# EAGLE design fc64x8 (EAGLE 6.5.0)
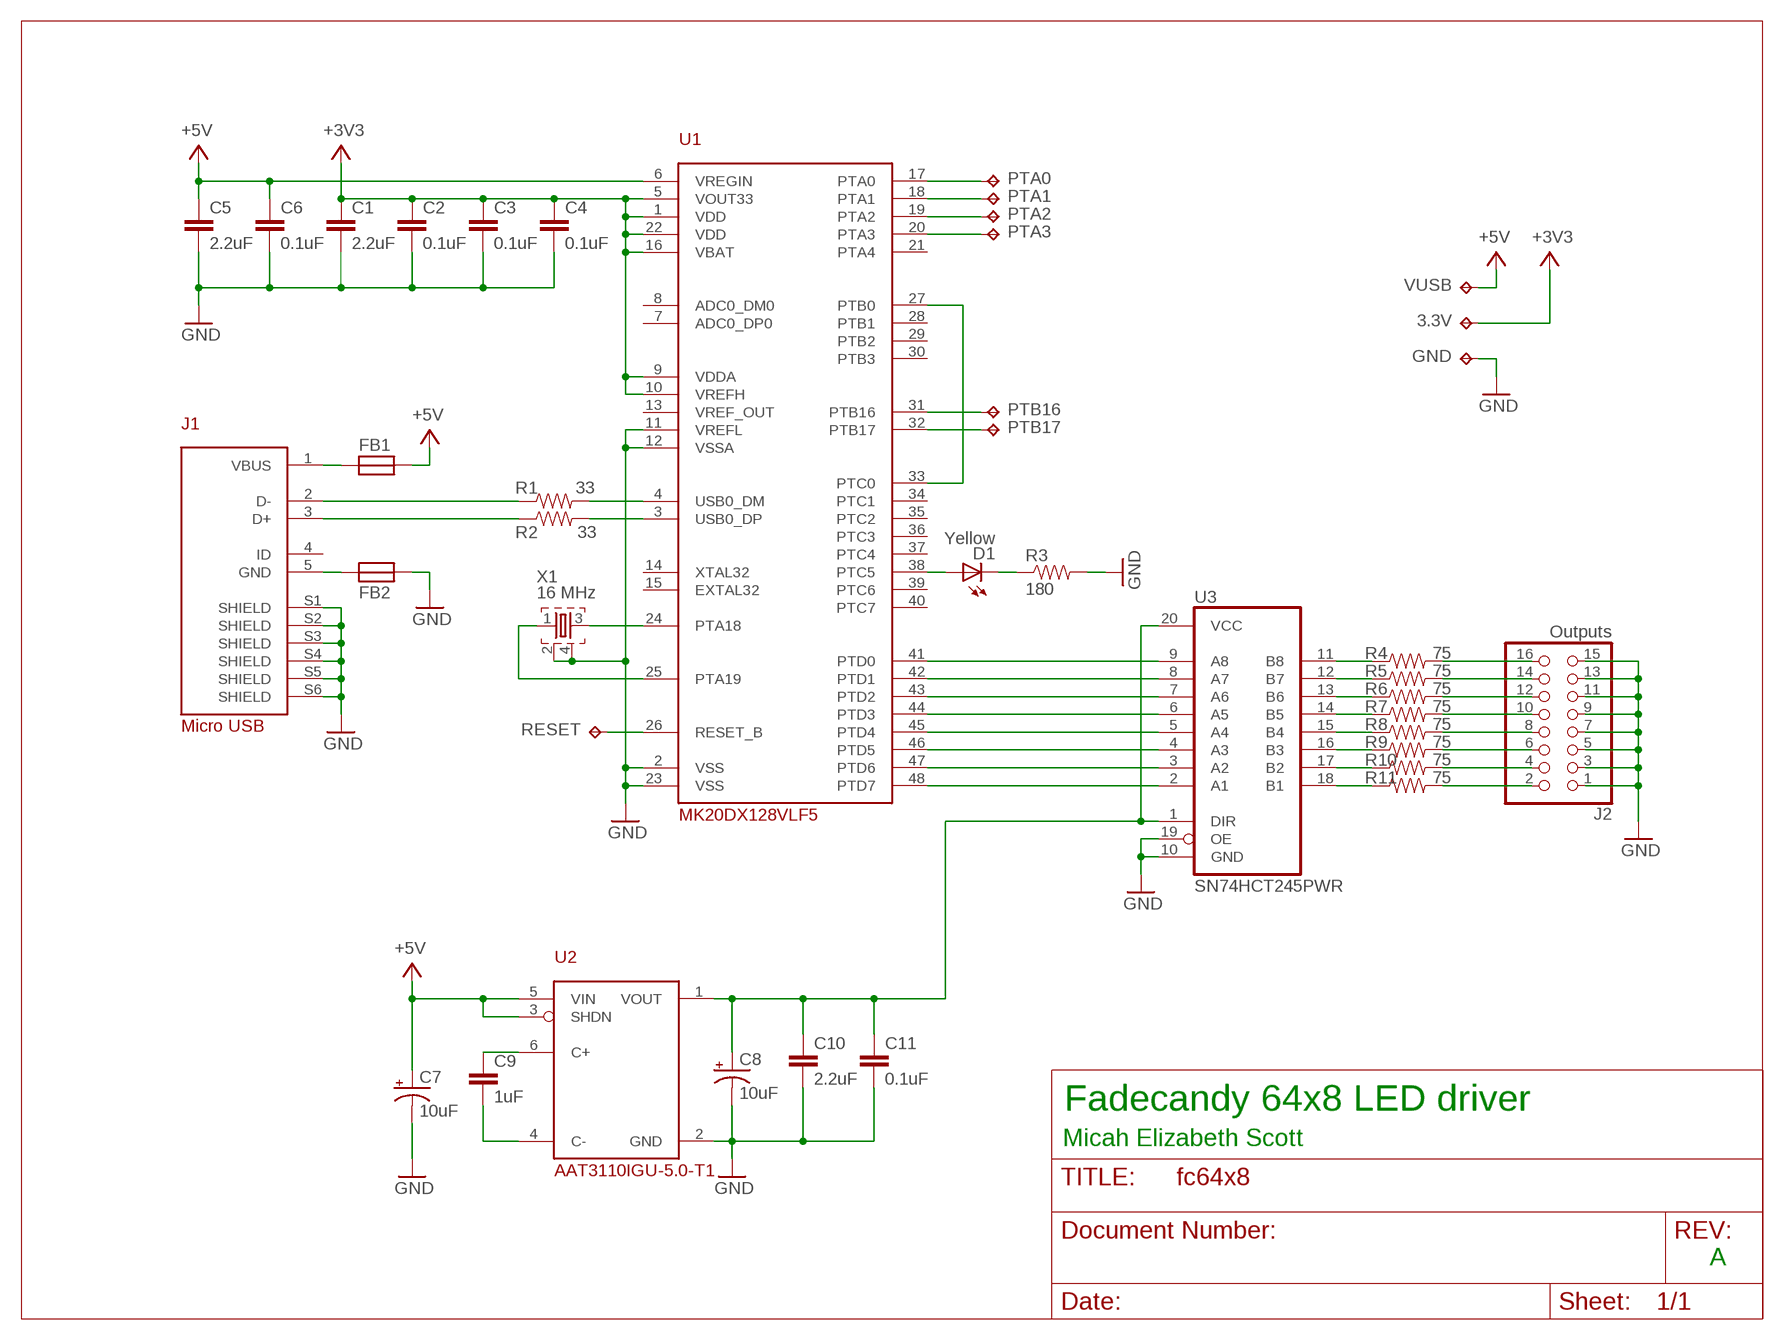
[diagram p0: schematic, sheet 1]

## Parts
3.3V  TPTP18SQ  [TP18SQ]
C1  2.2uF  CAP0603-CAP  [0603-CAP]
C2  0.1uF  CAP0603-CAP  [0603-CAP]
C3  0.1uF  CAP0603-CAP  [0603-CAP]
C4  0.1uF  CAP0603-CAP  [0603-CAP]
C5  2.2uF  CAP0603-CAP  [0603-CAP]
C6  0.1uF  CAP0603-CAP  [0603-CAP]
C7  10uF  CAP_POL1206  [EIA3216]
C8  10uF  CAP_POL1206  [EIA3216]
C9  1uF  CAP0603-CAP  [0603-CAP]
C10  2.2uF  CAP0603-CAP  [0603-CAP]
C11  0.1uF  CAP0603-CAP  [0603-CAP]
D1  Yellow  LED-YELLOW0603  [LED-0603]
FB1  FB  [0603]
FB2  FB  [0603]
GND  TPTP18SQ  [TP18SQ]
J1  Micro USB  USB-FCI-10118194  [FCI-10118194]
J2  Outputs  PINHD-2X8  [2X08]
PTA0  TPTP18SQ  [TP18SQ]
PTA1  TPTP18SQ  [TP18SQ]
PTA2  TPTP18SQ  [TP18SQ]
PTA3  TPTP18SQ  [TP18SQ]
PTB16  TPTP18SQ  [TP18SQ]
PTB17  TPTP18SQ  [TP18SQ]
R1  33  RESISTOR0603-RES  [0603-RES]
R2  33  RESISTOR0603-RES  [0603-RES]
R3  180  RESISTOR0603-RES  [0603-RES]
R4  75  RESISTOR0603-RES  [0603-RES]
R5  75  RESISTOR0603-RES  [0603-RES]
R6  75  RESISTOR0603-RES  [0603-RES]
R7  75  RESISTOR0603-RES  [0603-RES]
R8  75  RESISTOR0603-RES  [0603-RES]
R9  75  RESISTOR0603-RES  [0603-RES]
R10  75  RESISTOR0603-RES  [0603-RES]
R11  75  RESISTOR0603-RES  [0603-RES]
RESET  TPTP18SQ  [TP18SQ]
U1  MK20DX128VLF5  [LQFP48]
U2  AAT3110IGU-5.0-T1  AAT3110  [SOT23-6L]
U3  SN74HCT245PWR  74245PW  [TSSOP20]
VUSB  TPTP18SQ  [TP18SQ]
X1  16 MHz  TSX-32250  [TSX-3225]

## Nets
+3V3: 3.3V.TP C1.1 C2.1 C3.1 C4.1 U1.1(VDD) U1.5(VOUT33) U1.9(VDDA) U1.10(VREFH) U1.16(VBAT) U1.22(VDD)
+5V: C5.1 C6.1 C7.A(+) FB1.1 U1.6(VREGIN) U2.3(SHDN) U2.5(VIN) VUSB.TP
GND: C1.2 C2.2 C3.2 C4.2 C5.2 C6.2 C7.C(-) C8.C(-) C10.2 C11.2 FB2.1 GND.TP J1.S1(SHIELD) J1.S2(SHIELD) J1.S3(SHIELD) J1.S4(SHIELD) J1.S5(SHIELD) J1.S6(SHIELD) J2.1 J2.3 J2.5 J2.7 J2.9 J2.11 J2.13 J2.15 R3.2 U1.2(VSS) U1.11(VREFL) U1.12(VSSA) U1.23(VSS) U2.2(GND) U3.10(GND) U3.19(OE) X1.2 X1.4
N$1: D1.A U1.38(PTC5)
N$2: U1.24(PTA18) X1.3
N$3: D1.C R3.1
N$4: U1.25(PTA19) X1.1
N$5: FB1.2 J1.1(VBUS)
N$6: U1.27(PTB0) U1.33(PTC0)
N$7: FB2.2 J1.5(GND)
N$8: U1.41(PTD0) U3.9(A8)
N$9: J1.2(D-) R1.1
N$10: J1.3(D+) R2.1
N$11: R1.2 U1.4(USB0_DM)
N$12: R2.2 U1.3(USB0_DP)
N$13: U1.42(PTD1) U3.8(A7)
N$14: U1.43(PTD2) U3.7(A6)
N$15: U1.44(PTD3) U3.6(A5)
N$16: U1.45(PTD4) U3.5(A4)
N$17: U1.46(PTD5) U3.4(A3)
N$18: U1.47(PTD6) U3.3(A2)
N$19: U1.48(PTD7) U3.2(A1)
N$20: R4.1 U3.11(B8)
N$21: C9.1 U2.6(C+)
N$22: C9.2 U2.4(C-)
N$23: R5.1 U3.12(B7)
N$24: R6.1 U3.13(B6)
N$25: R7.1 U3.14(B5)
N$26: R8.1 U3.15(B4)
N$27: C8.A(+) C10.1 C11.1 U2.1(VOUT) U3.1(DIR) U3.20(VCC)
N$28: R9.1 U3.16(B3)
N$29: R10.1 U3.17(B2)
N$30: R11.1 U3.18(B1)
N$31: J2.16 R4.2
N$32: J2.14 R5.2
N$33: J2.12 R6.2
N$34: J2.10 R7.2
N$35: J2.8 R8.2
N$36: J2.6 R9.2
N$37: J2.4 R10.2
N$38: J2.2 R11.2
N$39: RESET.TP U1.26(RESET_B)
N$40: PTA0.TP U1.17(PTA0)
N$41: PTA1.TP U1.18(PTA1)
N$42: PTA2.TP U1.19(PTA2)
N$43: PTA3.TP U1.20(PTA3)
N$45: PTB16.TP U1.31(PTB16)
N$46: PTB17.TP U1.32(PTB17)
Unconnected: J1.4(ID) U1.7(ADC0_DP0) U1.8(ADC0_DM0) U1.13(VREF_OUT) U1.14(XTAL32) U1.15(EXTAL32) U1.21(PTA4) U1.28(PTB1) U1.29(PTB2) U1.30(PTB3) U1.34(PTC1) U1.35(PTC2) U1.36(PTC3) U1.37(PTC4) U1.39(PTC6) U1.40(PTC7)

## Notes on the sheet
- Fadecandy 64x8 LED driver
- Micah Elizabeth Scott
- A

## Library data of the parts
3.3V GND PTA0 PTA1-PTA3 PTB16 PTB17 RESET VUSB = testpad:TP: Test pad
C1-C6 C9-C11 = SparkFun-Passives:CAP: Capacitor
C7 C8 = SparkFun-Passives:CAP_POL: Capacitor Polarized
D1 = SparkFun-LED:LED-YELLOW: Yellow SMD LEDs; PROD_ID: DIO-09003
FB1 FB2 = scanlime:FB
J1 = scanlime:USB-FCI-10118194: Micro USB connector Digi-Key: 609-4618-1-ND
J2 = pinhead:PINHD-2X8: PIN HEADER
R1-R11 = SparkFun-Passives:RESISTOR: Resistor
U1 = scanlime:MK20DX128VLF5: ARM Cortex-M4 microcontroller with USB. Freescale K20 series 50 MHz 16 K RAM 128 K Flash Lower pincount equivalent to Teensy 3.0 2013 Price: $2.66 qty 100 Digi-Key: MK20DX128VLF50-ND
U2 = scanlime:AAT3110: Switched capacitor boost converter
U3 = scanlime:74*245: Octal BUS TRANSCEIVER, 3-state
X1 = scanlime:TSX-3225: MHz RANGE CRYSTAL UNIT Source: Epson Toyocom

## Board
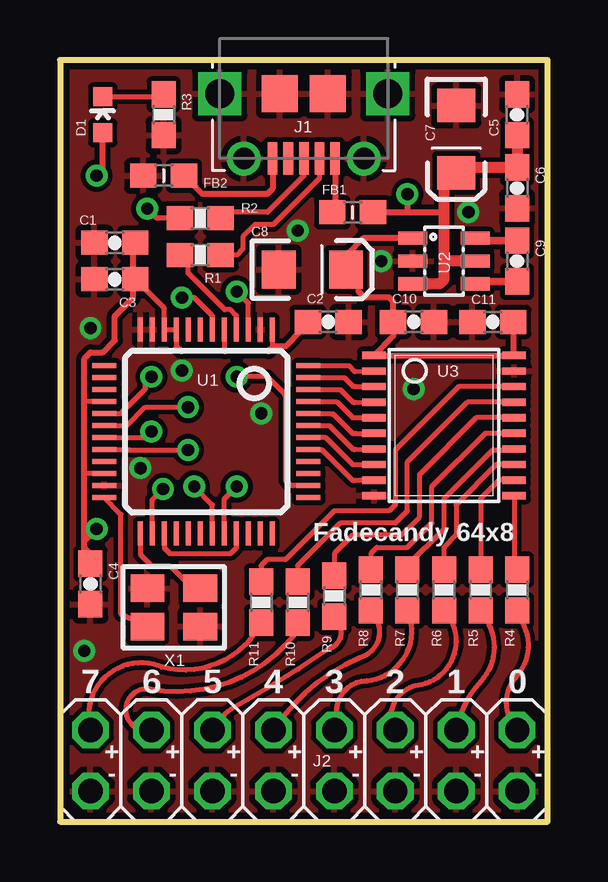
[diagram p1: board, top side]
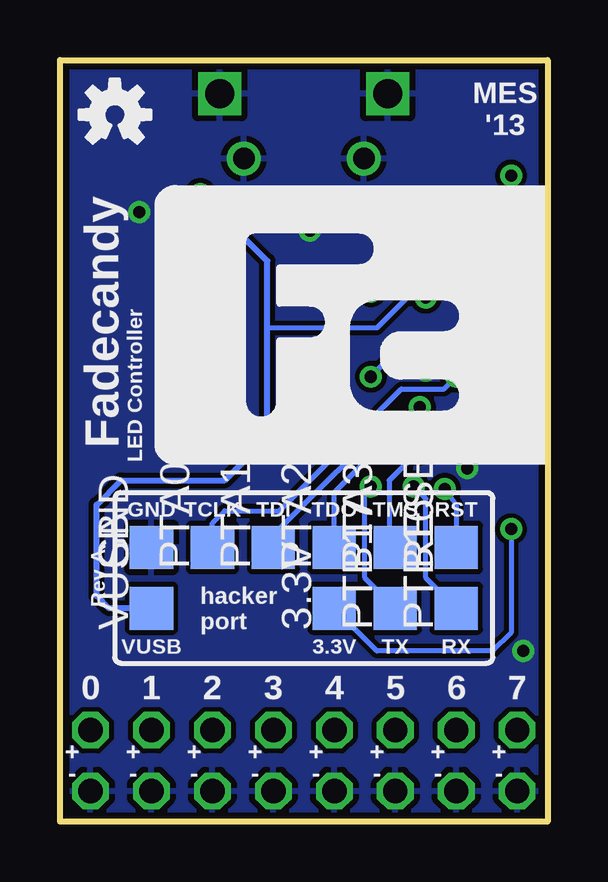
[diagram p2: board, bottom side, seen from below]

Size 20.32 x 31.75 mm. Coordinates in mm from the lower left corner, seen from the top.
Outline: 0,0 20.32,0 20.32,31.75 0,31.75 0,0
Copper layers (1*16): Top 0.035mm / dielectric 1.5mm / Bottom 0.035mm
Design rules "default *": minimum track width 8mil, minimum drill 20mil, track to track 8mil, track to pad 8mil, pad to pad 8mil, via to via 8mil, smd to smd 8mil, copper to edge 10mil, drill to drill 8mil, minimum pad ring 10mil, minimum via ring 8mil, stop-mask expansion 4mil, vias tented up to drill 25mil, thermal gap 10mil

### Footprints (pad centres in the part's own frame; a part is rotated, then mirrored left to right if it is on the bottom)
TP18SQ = smd 1.8 x 1.8: TP 0,0
0603-CAP = smd 1.1 x 1: 1 -0.85,0; 2 0.85,0
EIA3216 = smd 1.4 x 1.6: A 1.4,0; C -1.4,0
LED-0603 = smd 0.8 x 0.8: A 0,-0.75; C 0,0.75
0603 = smd 1.1 x 1: 1 -0.85,0; 2 0.85,0
FCI-10118194 = smd 0.4 x 1.35: 1 -1.3,0.3; 2 -0.65,0.3; 3 0,0.3; 4 0.65,0.3; 5 1.3,0.3 | drill 0.9: S1 -2.5,0.3; S2 2.5,0.3 | drill 1.2 square: S3 -3.5,-2.4; S4 3.5,-2.4 | smd 1.5 x 1.55: S5 -1,-2.4; S6 1,-2.4
2X08 = drill 1.016 octagon: 1 -8.89,-1.27; 2 -8.89,1.27; 3 -6.35,-1.27; 4 -6.35,1.27; 5 -3.81,-1.27; 6 -3.81,1.27; 7 -1.27,-1.27; 8 -1.27,1.27; 9 1.27,-1.27; 10 1.27,1.27; 11 3.81,-1.27; 12 3.81,1.27; 13 6.35,-1.27; 14 6.35,1.27; 15 8.89,-1.27; 16 8.89,1.27
0603-RES = smd 1.1 x 1: 1 -0.85,0; 2 0.85,0
LQFP48 = smd 0.203 x 1: 1 -2.75,-4.25; 2 -2.25,-4.25; 3 -1.75,-4.25; 4 -1.25,-4.25; 5 -0.75,-4.25; 6 -0.25,-4.25; 7 0.25,-4.25; 8 0.75,-4.25; 9 1.25,-4.25; 10 1.75,-4.25; 11 2.25,-4.25; 12 2.75,-4.25; 25 2.75,4.25; 26 2.25,4.25; 27 1.75,4.25; 28 1.25,4.25; 29 0.75,4.25; 30 0.25,4.25; 31 -0.25,4.25; 32 -0.75,4.25; 33 -1.25,4.25; 34 -1.75,4.25; 35 -2.25,4.25; 36 -2.75,4.25 | smd 1 x 0.203: 13 4.25,-2.75; 14 4.25,-2.25; 15 4.25,-1.75; 16 4.25,-1.25; 17 4.25,-0.75; 18 4.25,-0.25; 19 4.25,0.25; 20 4.25,0.75; 21 4.25,1.25; 22 4.25,1.75; 23 4.25,2.25; 24 4.25,2.75; 37 -4.25,2.75; 38 -4.25,2.25; 39 -4.25,1.75; 40 -4.25,1.25; 41 -4.25,0.75; 42 -4.25,0.25; 43 -4.25,-0.25; 44 -4.25,-0.75; 45 -4.25,-1.25; 46 -4.25,-1.75; 47 -4.25,-2.25; 48 -4.25,-2.75
SOT23-6L = smd 0.55 x 1.2: 1 -0.95,-1.3; 2 0,-1.3; 3 0.95,-1.3; 4 0.95,1.3; 5 0,1.3; 6 -0.95,1.3
TSSOP20 = smd 0.305 x 0.991: 1 -2.925,-2.918; 2 -2.275,-2.918; 3 -1.625,-2.918; 4 -0.975,-2.918; 5 -0.325,-2.918; 6 0.325,-2.918; 7 0.975,-2.918; 8 1.625,-2.918; 9 2.275,-2.918; 10 2.925,-2.918; 11 2.925,2.918; 12 2.275,2.918; 13 1.625,2.918; 14 0.975,2.918; 15 0.325,2.918; 16 -0.325,2.918; 17 -0.975,2.918; 18 -1.625,2.918; 19 -2.275,2.918; 20 -2.925,2.918
TSX-3225 = smd 1.4 x 1.15: 1 0,-1.6; 2 2.2,-1.6; 3 2.2,0; 4 0,0

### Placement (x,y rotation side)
3.3V  8.89,8.89 90 bottom
C1  2.29,24.13 180 top
C2  11.18,20.83 0 top
C3  2.29,22.61 180 top
C4  1.27,9.91 270 top
C5  19.05,29.46 90 top
C6  19.05,26.42 270 top
C7  16.51,28.45 270 top
C8  10.52,23.01 0 top
C9  19.05,23.37 270 top
C10  14.73,20.83 0 top
C11  18.03,20.83 180 top
D1  1.78,29.46 0 top
FB1  12.19,25.4 180 top
FB2  4.32,26.92 0 top
GND  16.51,11.43 90 bottom
J1  10.16,27.94 180 top
J2  10.16,2.54 0 top
PTA0  13.97,11.43 90 bottom
PTA1  11.43,11.43 90 bottom
PTA2  8.89,11.43 90 bottom
PTA3  6.35,11.43 90 bottom
PTB16  3.81,8.89 90 bottom
PTB17  6.35,8.89 90 bottom
R1  5.84,23.62 180 top
R2  5.84,25.15 180 top
R3  4.32,29.46 270 top
R4  19.05,9.65 270 top
R5  17.53,9.65 270 top
R6  16,9.65 270 top
R7  14.48,9.65 270 top
R8  12.95,9.65 270 top
R9  11.43,9.4 270 top
R10  9.91,9.14 270 top
R11  8.38,9.14 270 top
RESET  3.81,11.43 90 bottom
U1  6.1,16.26 180 top
U2  16,23.37 270 top
U3  16,16.51 270 top
U$1  [OSHW-LOGO-S]  18.03,29.46 0 bottom
VUSB  16.51,8.89 90 bottom
X1  5.84,8.13 180 top

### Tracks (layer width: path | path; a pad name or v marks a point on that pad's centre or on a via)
+3V3  (via drill 0.51)
  Top 0.203: 3.05,22.35 3.14,22.44 C3.1 4.35,21.4 U1.10 U1.9 4.85,19.79 | U1.22 1.04,14.51 1.02,14.48 | U1.16 1.04,17.51 1.02,17.53 | U1.1 8.85,19.77 8.89,19.81 | C4.1 1.27,11.18 1.02,11.43 1.02,11.68 v1.52,12.19 | U1.5 6.85,19.65 6.88,19.61
  Top 0.254: C4.1 1.02,10.92 1.02,11.43 1.02,14.48 1.02,17.53 1.02,19.3 1.27,19.56 1.78,19.56 2.29,20.07 2.29,21.08 3.05,21.84 3.05,22.35 3.05,24.3 C1.1 | 4.85,19.79 5.05,19.61 6.88,19.61 8.69,19.61 8.85,19.77 | C2.1 10.07,20.49 9.4,19.81 8.89,19.81
  Bottom 0.203: v1.52,12.19 1.52,7.87 2.29,7.11 7.11,7.11 3.3V.TP
+5V  (via drill 0.51)
  Top 0.203: U1.6 6.35,21.09 5.59,21.84 v5.08,21.84
  Top 0.254: 16.73,27.27 C7.A 16,27.05 | FB1.1 14.48,25.4 | 14.48,25.4 16,25.4 | v14.48,26.16 14.48,25.4
  Top 0.457: C5.1 C6.1 16.73,27.27 | U2.3 15.81,22.42 16,22.61 16,23.37 | 16,23.37 16,25.4 16,27.05 | U2.5 16,23.37
  Bottom 0.203: v5.08,21.84 5.84,21.84 7.11,20.57 11.68,20.57
  Bottom 0.254: VUSB.TP 18.29,8.89 18.8,9.4 18.8,13.21 17.78,14.22 13.46,14.22 11.68,16 11.68,20.57 11.68,23.37 v14.48,26.16
GND  (via drill 0.51)
  other vias: 1.02,7.11 14.73,18.03 8.38,17.02 1.27,20.57 13.39,23.37 9.91,24.64 3.35,14.73 5.08,18.8 17.02,25.4
  pour Bottom: 0,31.75 20.32,31.75 20.32,0 0,0
  pour Top: 0,31.75 20.32,31.75 20.32,0 0,0
N$1  (via drill 0.51)
  Top 0.203: 1.78,27.28 arc-45 1.7,27.1 v1.52,26.92 | U1.38 9.72,14.01 arc-45 9.54,14.08 9.4,14.22 9.4,17.68 arc45 9.32,17.85 8.64,18.54 v7.37,18.54
  Top 0.254: 1.78,27.28 D1.A
  Bottom 0.203: v7.37,18.54 5.84,20.07 3.3,20.07 2.54,20.83 2.54,23.88 1.52,24.89 v1.52,26.92
N$2
  Top 0.203: X1.3 2.54,8.64 2.54,12.81 U1.24
N$3
  Top 0.203: D1.C 4.11,30.21 arc45 4.29,30.29 R3.1
N$4
  Top 0.203: U1.25 3.35,11.13 3.81,10.67 4.57,10.67 5.33,9.91 X1.1
N$5
  Top 0.254: J1.1 11.46,25.77 FB1.2
N$6
  Top 0.203: U1.27 4.35,11.4 4.57,11.18 7.11,11.18 7.35,11.41 U1.33
N$7
  Top 0.254: J1.5 8.86,26.39 8.64,26.16 5.93,26.16 FB2.2
N$8
  Top 0.203: 12.45,14.22 U3.9 12.31,14.22 12.19,14.22 10.91,15.51 U1.41
N$9
  Top 0.203: J1.2 10.81,26.81 8.89,24.89 8.13,24.89 7.62,24.38 7.62,23.88 7.37,23.62 R1.1
N$10
  Top 0.203: J1.3 10.16,26.92 8.64,25.4 6.95,25.4 R2.1
N$11
  Top 0.203: U1.4 7.35,21.1 7.11,21.34 6.86,21.34 5.33,22.86 5.33,23.28 R1.2
N$12  (via drill 0.51)
  Top 0.203: U1.3 7.85,21.62 v7.37,22.1 | R2.2 4.04,25.15 v3.63,25.55
  Bottom 0.203: v7.37,22.1 v3.63,25.55
N$13
  Top 0.203: 10.66,16.01 U1.42 11.07,16 12.19,14.88 12.32,14.88 U3.8
N$14
  Top 0.203: U1.43 10.66,16.51 10.92,16.51 11.23,16.51 12.22,15.52 12.31,15.52 U3.7
N$15
  Top 0.203: U1.44 11.26,17.01 11.28,16.99 11.38,16.99 12.19,16.18 12.32,16.18 U3.6
N$16
  Top 0.203: U1.45 11.53,17.51 12.19,16.84 12.32,16.84 U3.5
N$17
  Top 0.203: U1.46 11.69,18.01 12.22,17.48 12.31,17.48 U3.4
N$18
  Top 0.203: U1.47 11.85,18.51 12.22,18.14 12.32,18.14 U3.3
N$19
  Top 0.203: U1.48 12.03,19.01 12.27,18.77 12.31,18.77 U3.2
N$20
  Top 0.203: U3.11 18.92,10.63 R4.1
N$21
  Top 0.254: 17.4,24.22 U2.6
  Top 0.305: 17.4,24.22 C9.1
N$22
  Top 0.254: 17.4,22.52 U2.4
  Top 0.305: 17.4,22.52 C9.2
N$23
  Top 0.203: U3.12 18.3,14.23 17.53,13.46 R5.1
N$24
  Top 0.203: R6.1 16,11.43 16.51,11.94 16.51,13.21 18.19,14.88 U3.13
N$25
  Top 0.203: R7.1 14.48,10.67 16,12.19 16,13.46 18.03,15.49 18.88,15.49 U3.14
N$26
  Top 0.203: U3.15 17.71,16.18 15.49,13.97 15.49,12.45 14.48,11.43 13.21,11.43 12.95,11.18 R8.1
N$27
  Top 0.254: U2.1 12.63,24.32 11.94,23.62 C8.A 12.45,22.74 12.45,22.1 12.7,21.84 13.72,21.84 13.88,21.68 C10.1 13.88,20.23 U3.1 U3.20 18.88,19.47 C11.1
N$28
  Top 0.203: U3.16 17.34,16.84 14.99,14.48 14.99,12.7 14.22,11.94 12.19,11.94 11.43,11.18 R9.1
N$29
  Top 0.203: U3.17 16.98,17.48 14.48,14.99 14.48,12.95 13.97,12.45 11.68,12.45 9.91,10.67 R10.1
N$30
  Top 0.203: U3.18 16.61,18.14 13.97,15.49 13.97,13.21 13.72,12.95 11.43,12.95 9.4,10.92 8.64,10.92 8.38,10.67 R11.1
N$31
  Top 0.203: R4.2 19.18,8.43 arc-75 19.05,6.1 arc88 J2.16
N$32
  Top 0.203: R5.2 17.78,8.38 arc-74 17.53,5.84 arc32 J2.14
N$33
  Top 0.203: J2.12 13.79,4.45 arc-80 15.06,5.71 arc121 R6.2
N$34
  Top 0.203: J2.10 11.53,4.6 arc-90 12.8,5.87 arc108 R7.2
N$35
  Top 0.203: R8.2 13.21,8.38 arc-99 12.5,6.83 arc33 J2.8
N$36
  Top 0.203: R9.2 11.28,8.56 arc-140 11.18,7.19 arc-5 7.37,4.83 arc34 J2.6
N$37
  Top 0.203: R10.2 10.06,8.2 arc-67 3.79,5.51 arc205 J2.4
N$38
  Top 0.203: R11.2 8.13,7.87 arc-77 3.91,6.55 arc120 J2.2
N$39  (via drill 0.51)
  Top 0.203: U1.26 3.85,13.42 v4.29,13.87
  Bottom 0.203: v4.29,13.87 3.81,13.21 RESET.TP
N$40  (via drill 0.51)
  Top 0.203: U1.17 2.53,17.01 3.56,18.03 3.56,18.29 v3.81,18.54
  Bottom 0.203: PTA0.TP 13.97,12.45 13.46,12.95 11.18,12.95 6.1,18.03 4.32,18.03 v3.81,18.54
N$41  (via drill 0.51)
  Top 0.203: U1.18 arc45 U1.18 2.79,16.51 3.56,17.27 v5.33,17.27
  Bottom 0.203: PTA1.TP 11.43,12.19 11.18,12.19 6.35,17.02 5.59,17.02 v5.33,17.27
N$42  (via drill 0.51)
  Top 0.203: U1.19 arc45 U1.19 3.56,16 v3.81,16.26
  Bottom 0.203: PTA2.TP 8.89,13.72 6.35,16.26 v3.81,16.26
N$43  (via drill 0.51)
  Top 0.203: v5.33,15.49 2.64,15.49 2.88,15.51 U1.20
  Bottom 0.203: v5.33,15.49 6.6,14.22 6.6,11.68 PTA3.TP
N$45  (via drill 0.51)
  Top 0.203: U1.31 6.35,13.2 v5.59,13.97
  Bottom 0.203: PTB16.TP 5.08,10.16 5.08,13.46 v5.59,13.97
N$46  (via drill 0.51)
  Top 0.203: U1.32 6.85,13.45 v7.37,13.97
  Bottom 0.203: PTB17.TP 7.62,10.16 7.62,13.72 v7.37,13.97

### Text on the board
tPlace: Fadecandy 64x8 | 7 | 6 | 5 | 4 | 3 | 2 | 1 | 0 | + | + | + | + | + | + | + | + | - | - | - | - | - | - | - | -
bPlace: MES / '13 | Fadecandy | LED Controller | RST | TMS | TDO | TDI | TCLK | GND | Rev A | hacker / port | RX | TX | 3.3V | VUSB | 7 | 6 | 5 | 4 | 3 | 2 | 1 | 0 | + | + | + | + | + | + | + | + | - | - | - | - | - | - | - | -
